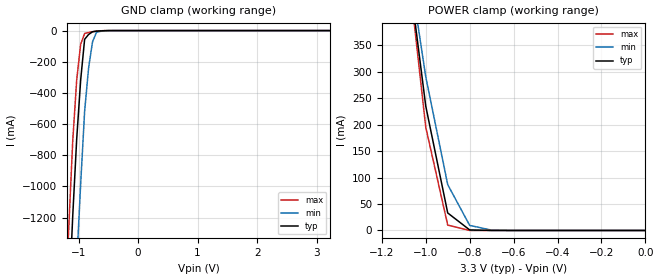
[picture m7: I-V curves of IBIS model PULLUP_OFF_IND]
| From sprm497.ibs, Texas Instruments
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|   Model Cell PULLUP_OFF_IND
[Model]   PULLUP_OFF_IND
Model_type   Input
Polarity   Non-Inverting
Vinl =  0.8
Vinh =  2
C_comp   0.8695239p   0.8584917p   0.8767336p
[Model Spec]
Vinl   0.8   0.8   0.8
Vinh   2   2   2
[Temperature Range]   25   125   -40
[Voltage Range]   3.3   3.14   3.47
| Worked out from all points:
|   GND clamp passes 1 mA (typ) near -0.58 V on its own axis
|   POWER clamp passes 1 mA (typ) near -0.80 V on its own axis
[POWER_clamp]
|   voltage   I(typ)   I(min)   I(max)
-3.3V     9.572A     8.116A     10.87A
-1.067V   452.2mA    472.9mA    444.7mA
-1.033V   343.6mA    381.6mA    319.9mA
-1V       234.9mA    290.3mA    195.1mA
-900mV    33.06mA    86.54mA    10.16mA
-800mV    1.024mA    9.598mA    94.09uA
-700mV    26.08uA    628.6uA    3.452uA
-11.55fV  365.2pA    11.75nA    167pA
[GND_clamp]
|   voltage   I(typ)   I(min)   I(max)
-3.3V     -22.43A    -23.21A    -22A
-1.233V   -2.35A     -3.221A    -1.845A
-1.167V   -1.763A    -2.627A    -1.266A
-1.1V     -1.191A    -2.042A    -709.2mA
-1.033V   -696.7mA   -1.494A    -318mA
-966.7mV  -318.5mA   -986.5mA   -87.78mA
-900mV    -56.13mA   -518.4mA   -18.69mA
-833.3mV  -25.12mA   -240.3mA   -12.29mA
-766.7mV  -7.66mA    -71.22mA   -7.13mA
-700mV    -3.748mA   -11.19mA   -3.213mA
-433.3mV  -54.28uA   -212.3uA   -16.6uA
3.233V    344.9pA    12.54nA    142.7pA
